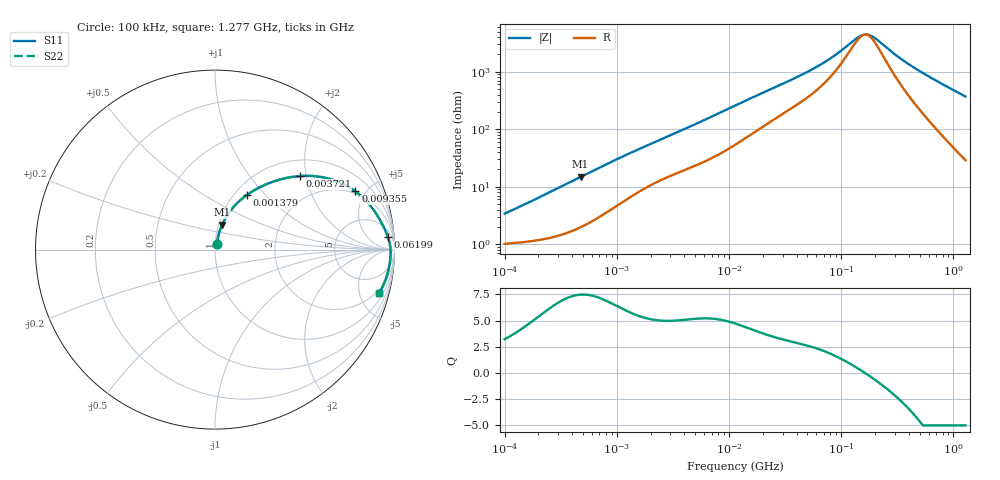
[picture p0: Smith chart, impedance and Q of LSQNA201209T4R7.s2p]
! LSQNA201209T4R7  S-PARAMETER MODEL  ( General Type )
! Model Generated by TAIYO YUDEN Corporation (http://www.ty-top.com)
! Version 2.0
! TAIYO YUDEN Control No. 100810NF25SB-FKC
! Copyright(c) 2007 TAIYO YUDEN CO.,LTD. All Rights Reserved.
! Product Description (link to TY-COMPAS)
! https://ds.yuden.co.jp/TYCOMPAS/or/detail?pn=LSQNA201209T4R7M&u=M
! Products Name : Inductors
! Characteristics :
!  Inductance : 4.7 uH , SRF(min) : 45 MHz , DC Resistance(max) : 0.858 Ohm
!  Rated Current : Saturation :275 mA , Temp Rise : 490 mA (40 degC)
!  Case Size : 2.0 x 1.25 / 0.079 x 0.049 [mm/inch] , Thickness : 0.9 / 0.035 [mm/inch]
!  (Conditions: Temperature = 25 degC , DC Bias Current/Voltage = 0A / 0V)
! External Node Assignments :
!  1  o---GGG---o  2
! GND o---------o GND
! Frequency Range : 0.1MHz  -  1277.432519MHz  [ 402 STEP ]
# MHz S RI R 50
! Freq[MHz].  S11 Real  S11 Imag  S21 Real  S21 Imag  S12 Real  S12 Imag  S22 Real  S22 Imag
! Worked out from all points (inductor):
!   401 points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, 100 kHz to 1.277 GHz, reference 50 ohm
!   read as one part in series: L = 5.1 uH near 104.8 kHz
!   highest Q = 7.47 at 475.9 kHz (marker M1), where L = 4.92 uH
!   self-resonance near 163.1 MHz
!   S11 on the Smith chart (normalised r, x): 100 kHz: 1.02, +0.07; 1.379 MHz: 1.14, +0.79; 3.721 MHz: 1.37, +1.84; 9.355 MHz: 1.85, +4.24; 61.99 MHz: 11, +23; 1.277 GHz: 1.58, -7.41
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0.1  0.011 0.0318  0.989 -0.0318  0.989 -0.0318  0.011 0.0318
0.234191  0.0175 0.0715  0.9825 -0.0715  0.9825 -0.0715  0.0175 0.0715
0.475933  0.0394 0.1387  0.9606 -0.1387  0.9606 -0.1387  0.0394 0.1387
0.487317  0.0407 0.1417  0.9593 -0.1417  0.9593 -0.1417  0.0407 0.1417
0.839317  0.0899 0.2217  0.9101 -0.2217  0.9101 -0.2217  0.0899 0.2217
1.378824  0.1773 0.3039  0.8227 -0.3039  0.8227 -0.3039  0.1773 0.3039
2.374779  0.3223 0.3781  0.6777 -0.3781  0.6777 -0.3781  0.3223 0.3781
3.721125  0.4741 0.4099  0.5259 -0.4099  0.5259 -0.4099  0.4741 0.4099
5.694551  0.6298 0.3963  0.3702 -0.3963  0.3702 -0.3963  0.6298 0.3963
9.354966  0.7818 0.3246  0.2182 -0.3246  0.2182 -0.3246  0.7818 0.3246
11.5727  0.8284 0.2851  0.1716 -0.2851  0.1716 -0.2851  0.8284 0.2851
21.3967  0.9094 0.1814  0.0906 -0.1814  0.0906 -0.1814  0.9094 0.1814
55.07831  0.9607 0.0782  0.0393 -0.0782  0.0393 -0.0782  0.9607 0.0782
61.98831  0.9643 0.0684  0.0357 -0.0684  0.0357 -0.0684  0.9643 0.0684
88.3685  0.9721 0.0414  0.0279 -0.0414  0.0279 -0.0414  0.9721 0.0414
138.4677  0.9772 0.0107  0.0228 -0.0107  0.0228 -0.0107  0.9772 0.0107
159.5672  0.9779 0.00143  0.0221 -0.00143  0.0221 -0.00143  0.9779 0.00143
175.3909  0.9782 -0.00481  0.0218 0.00481  0.0218 0.00481  0.9782 -0.00481
192.7837  0.9784 -0.0111  0.0216 0.0111  0.0216 0.0111  0.9784 -0.0111
268.406  0.978 -0.0345  0.022 0.0345  0.022 0.0345  0.978 -0.0345
508.1244  0.9709 -0.0925  0.0291 0.0925  0.0291 0.0925  0.9709 -0.0925
1277.433  0.9162 -0.2408  0.0838 0.2408  0.0838 0.2408  0.9162 -0.2408
